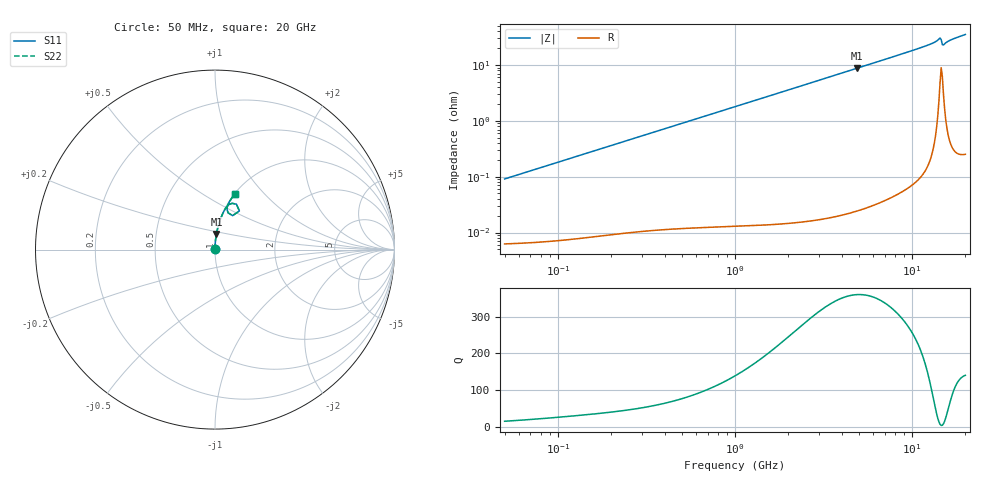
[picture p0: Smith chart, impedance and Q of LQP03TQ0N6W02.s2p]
!Murata Part Number: LQP03TQ0N6W02
!These Parameters are Measured in Series Mode Connection
!  o--[Z]--o
!Port1  Port2
!  o-------o
!Freq. Start=50[MHz] Stop=20[GHz], 401[Steps]
# Hz S RI R 50
!Freq.(Hz) S11(Real) S11(Imag) S21(Real) S21(Imag) S12(Real) S12(Imag) S22(Real) S22(Imag)
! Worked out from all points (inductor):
!   401 points, 50 MHz to 20 GHz, reference 50 ohm
!   read as one part in series: L = 289 pH near 51.52 MHz
!   highest Q = 361 at 4.893 GHz (marker M1), where L = 285 pH
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5e7  6.33e-05 0.000908  0.9999 -0.000908  0.9999 -0.000908  6.33e-05 0.000908
5.152053e7  6.35e-05 0.000936  0.9999 -0.000936  0.9999 -0.000936  6.35e-05 0.000936
1.364002e8  8.51e-05 0.00247  0.9999 -0.00247  0.9999 -0.00247  8.51e-05 0.00247
3.721004e8  0.000155 0.00667  0.9998 -0.00667  0.9998 -0.00667  0.000155 0.00667
1e9  0.000448 0.0179  0.9996 -0.0179  0.9996 -0.0179  0.000448 0.0179
1.714689e9  0.00108 0.0306  0.9989 -0.0306  0.9989 -0.0306  0.00108 0.0306
2.728004e9  0.00253 0.0486  0.9975 -0.0486  0.9975 -0.0486  0.00253 0.0486
4.89267e9  0.00785 0.0869  0.9921 -0.0869  0.9921 -0.0869  0.00785 0.0869
7.442007e9  0.018 0.1313  0.982 -0.1313  0.982 -0.1313  0.018 0.1313
9.600142e9  0.0299 0.1684  0.9701 -0.1684  0.9701 -0.1684  0.0299 0.1684
1.201863e10  0.0479 0.2104  0.9521 -0.2104  0.9521 -0.2104  0.0479 0.2104
1.334722e10  0.064 0.237  0.936 -0.237  0.936 -0.237  0.064 0.237
1.396067e10  0.0816 0.2529  0.9184 -0.2529  0.9184 -0.2529  0.0816 0.2529
1.417136e10  0.0952 0.2577  0.9048 -0.2577  0.9048 -0.2577  0.0952 0.2577
1.460232e10  0.1358 0.2155  0.8642 -0.2155  0.8642 -0.2155  0.1358 0.2155
1.504638e10  0.0737 0.2044  0.9263 -0.2044  0.9263 -0.2044  0.0737 0.2044
1.527346e10  0.0677 0.2199  0.9323 -0.2199  0.9323 -0.2199  0.0677 0.2199
1.550395e10  0.0673 0.231  0.9327 -0.231  0.9327 -0.231  0.0673 0.231
1.597544e10  0.0709 0.2462  0.9291 -0.2462  0.9291 -0.2462  0.0709 0.2462
1.670968e10  0.0781 0.2623  0.9219 -0.2623  0.9219 -0.2623  0.0781 0.2623
1.855685e10  0.0971 0.2923  0.9029 -0.2923  0.9029 -0.2923  0.0971 0.2923
2e10  0.1123 0.3122  0.8877 -0.3122  0.8877 -0.3122  0.1123 0.3122
